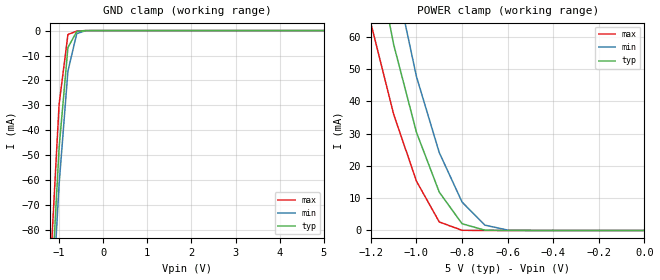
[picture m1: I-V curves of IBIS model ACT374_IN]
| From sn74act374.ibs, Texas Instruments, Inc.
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|   Model ACT374_IN
[Model]   ACT374_IN
Model_type  Input
Polarity   Non-Inverting
Vinl = 0.8
Vinh = 2.0
| variable   typ   min   max
C_comp   2.5pF   NA   NA
[Temperature Range]   40   100   -40
| Ambient temperature   25   85   -40
[Voltage range]   5.0   4.5   5.5
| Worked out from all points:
|   GND clamp passes 1 mA (typ) near -0.62 V on its own axis
|   POWER clamp passes 1 mA (typ) near -0.75 V on its own axis
[GND Clamp]
|   Voltage   I(typ)   I(min)   I(max)
-5V       -1.852A    -1.655A    -2.072A
-1.2V     -113.2mA   -124.5mA   -95.91mA
-1V       -46.97mA   -61.63mA   -29.6mA
-800mV    -6.816mA   -16.26mA   -1.572mA
-600mV    -356.6uA   -1.222mA   -210uA
-400mV    -15.11uA   -55.41uA   -1.392uA
5V        104.2pA    153.3pA    26.02pA
[POWER Clamp]
|   Voltage   I(typ)   I(min)   I(max)
-5V       2.785A     2.585A     3.504A
-1.2V     93.62mA    117.7mA    64.15mA
-1.1V     57.56mA    80.78mA    35.95mA
-1V       30.37mA    47.62mA    15.25mA
-900mV    11.87mA    24.11mA    2.641mA
-800mV    2.088mA    8.807mA    49.48uA
-700mV    89.92uA    1.657mA    385.9nA
-600mV    2.014uA    120.7uA    2.899nA
0V        979.8pA    374pA      36.08pA
